(* Logix 5000 AddOnInstructionDefinition export AOI_MOXA_SWITCH_28P_v1_1; software revision 20.01 *)

TYPE MOXA_Ethernet_Link_Object :   // class 0xf6
STRUCT
   Interface_Speed : DINT;   // Interface speed currently in use. Speed in Mbps (e.g., 0, 10, 100, 1000, etc.)
   Interface_Flags : MOXA_Interface_Object_Flags;   // Interface status flags
   Physical_Address : SINT[6];   // MAC layer address
   InOctets : DINT;   // Octets received on the interface
   InUcastPackets : DINT;   // Unicast packets received on the interface
   InNucastPackets : DINT;   // Non-unicast packets received on the interface
   InDiscards : DINT;   // Inbound packets received on the interface but discarded
   InErrors : DINT;   // Inbound packets that contain errors (does not include In Discards)
   InUnknownProtos : DINT;   // Inbound packets with unknown protocol.
   OutOctets : DINT;   // Octets sent on the interface
   OutUcastPackets : DINT;   // Unicast packets sent on the interface
   OutNucastPackets : DINT;   // Non-unicast packets sent on the interface
   OutDiscards : DINT;   // Outbound packets discarded
   OutErrors : DINT;   // Outbound packets that contain errors
   Alignment_Errors : DINT;   // Frames received that are not an integral number of octets in length
   FCS_Errors : DINT;   // Frames received that do not pass the FCS check
   Single_Collisions : DINT;   // Successfully transmitted frames which experienced exactly one collision
   Multiple_Collisions : DINT;   // Successfully transmitted frames which experienced more than one collision
   SQE_Test_Errors : DINT;   // Number of times SQE test error message is generated
   Deferred_Transmissions : DINT;   // Frames for which first transmission attempt is delayed because the medium is busy
   Late_Collisions : DINT;   // Number of times a collision is detected later than 512 bit- times into the transmission of a packet
   Excessive_Collisions : DINT;   // Frames for which transmission fails due to excessive collisions
   MAC_Transmit_Errors : DINT;   // Frames for which transmission fails due to an internal MAC sublayer transmit error
   Carrier_Sense_Errors : DINT;   // Times that the carrier sense condition was lost or never asserted when attempting to transmit a frame
   Frame_Too_Long : DINT;   // Frames received tha exceed the maximum permitted frame size.
   MAC_Receive_Errors : DINT;   // Frames for which reception on an interface fails due to an internal MAC sublayer receive error
   Control_Bits : INT;   // Bit 0 Auto-negotiate Bit 1: Forced Duplex Mode Bit 2-15: Reserved.
   Forced_Interface_Speed : INT;   // Speed at which the interface shall be forced to operate. Speed in Mbps (10, 100, 1000, etc.)
   Interface_Label : STRING;   // Port Description
   Capability_Bits : DINT;
   Speed_Duplex_Array : SINT;   // Number of elements
   Interface_Speed_Duplex_Capbility : MOXA_Interface_Capability[4];
   HC_InOctets : LINT;   // The total number of octets received on the interface. This counter is a 64-bit version of In Octets.
   HC_InUcastPkts : LINT;   // Unicast packets received on the interface. This counter is a 64-bit version of In Ucast Packets.
   HC_InMulticastPkts : LINT;   // Multicast packets received on the interface.
   HC_InBroadcastPkts : LINT;   // Broadcast packets received on the interface.
   HC_OutOctets : LINT;   // Octets sent on the interface. This counter is a 64-bit version of Out Octets.
   HC_OutUcastPkts : LINT;   // Unicast packets sent on the interface. This counter is a 64-bit version of Out Ucast Packets.
   HC_OutMulticastPkts : LINT;   // Multicast packets sent on the interface.
   HC_OutBroadcastPkts : LINT;   // Broadcast packets sent on the interface.
   HC_StatsAlignmentErrors : LINT;   // Frames received that are not an integral number of octets in length and do not pass the FCS check. This counter is a 64-bit version of Alignment Errors.
   HC_StatsFCSErrors : LINT;   // Frames received that are an integral number of octets in length but do not pass the FCS check. This counter is a 64-bit version of FCS Errors.
   HC_StatsInternalMacTransmitErrors : LINT;   // Frames for which transmission fails due to an internal MAC sublayer transmit error. This counter is a 64-bit version of MAC Transmit Errors.
   HC_StatsFrameTooLongs : LINT;   // Frames received that exceed the maximum permitted frame size. This counter is a 64-bit version of Frame Too Long Errors.
   HC_StatsInternalMacReceiveErrors : LINT;   // Frames for which reception on an interface fails due to an internal MAC sublayer receive error. This counter is a 64-bit version of MAC Receive Errors.
   HC_StatsSymbolErrors : LINT;   // Number of times there was an invalid data symbol on the media when a valid carrier was present.
   Port_State : SINT;   // Switch port state. Value 1 = Disable Value 2 = Blocking Value 3 = Listening Value 4 = Learning Value 5 = Forwarding Value 6 = Broken
   Media_Type : STRING;   // Port media type. Ex: "1000TX,RJ45"
   Traffic_Storm_Control : SINT;   // Traffic storm control enable. Bit 0: Broadcast storm control Bit 1: Multicast storm control Bit 2: DLF storm control
   Port_On_Event : SINT;   // Registered port for port on event notification. 0 = Unregistered. 1 = Registered.
   Port_Off_Event : SINT;   // Registered port for port off event notification. 0 = Unregistered. 1 = Registered.
   Port_Shutdown_by_PSEC_Event : SINT;   // Registered port for port shut down by Port Security event notification. 0 = Unregistered. 1 = Registered.
   Port_Shutdown_by_Rate_Limit_Event : SINT;   // Registered port for port shut down by Rate Limit event notification. 0 = Unregistered. 1 = Registered.
   Port_Recovered_by_Rate_Limit_Event : SINT;   // Registered port for port recovered by Rate Limit event notification. 0 = Unregistered. 1 = Registered.
   Fiber_Check_Warning_Event : SINT;   // Registered port for fiber check warning event notification. 0 = Unregistered. 1 = Registered.
END_STRUCT
END_TYPE

TYPE MOXA_TCPIP_Interface_Object :   // class 0xf5
STRUCT
   Status : DINT; {access Read Only}   // Interface Status
   Configuration_Capability : DINT;   // Interface capability flags
   Configuration_Control : DINT;   // Interface control flags
   Path_Size : INT;   // Size of Path
   Object_Path : DINT;   // Logical segments identifying the physical link object
   IP_Address : DINT;   // The device’s IP address.
   Network_Mask : DINT;   // The device’s network mask
   Gateway_Address : DINT;   // Default gateway address
   Name_Server_1 : DINT;   // Primary name server
   Name_Server_2 : DINT;   // Secondary name server
   Domain_Name : STRING;   // Default domain name
   Host_Name : STRING;   // Host Name
   Encapsulation_InactivityTimeout : INT;   // Number of seconds of inactivity before TCP connection is closed.
END_STRUCT
END_TYPE

TYPE MOXA_Interface_Capability :   // Indication of capabilities of the interface
STRUCT
   Interface_Speed_Capbility : INT;   // Interface speed currently in use. Speed in Mbps (e.g., 0, 10, 100, 1000, etc.)
   Interface_Duplex_Mode : SINT;   // 0=half duplex, 1=full duplex
END_STRUCT
END_TYPE

TYPE MOXA_String_32 :   // string type; Display the ip address, network mask, MAC address
STRUCT
   LEN : DINT;
   DATA : SINT[32];
END_STRUCT
END_TYPE

TYPE MOXA_HMI_Set_Object :
STRUCT
   Select_Port : INT;   // current port select on FT View
   Reset_to_default : SINT;   // Reboot and reset to default. 0 = Reserved. 1 = Reboot the device 2 = Reset to default
   Reset_MIB_Counter : SINT;   // Reset MIB counters. Any value indicates to reset port MIB counter.
   Speed_Duplex : SINT;
   Enter_Port_Setting : BOOL;   // Ready for port setting
   Enter_Reset_Setting : BOOL;   // Ready for resetting.
END_STRUCT
END_TYPE

TYPE MOXA_Interface_Object_Flags :   // reference to Ethernet Link object
STRUCT
   Link_Status : BOOL;   // 0-inactive, 1-active
   Duplex : BOOL;   // 0-half, 1-full
   Negotiation_Status_1 : BOOL;
   Negotiation_Status_2 : BOOL;
   Negotiation_Status_3 : BOOL;
   Manual_Setting_Requires_Reset : BOOL;
   Local_Hardware_Fault : BOOL;
END_STRUCT
END_TYPE

TYPE MOXA_Base_Switch_Object :   // calss 0x51
STRUCT
   Device_Up_Time : DINT;   // Time since device was powered up.
   Total_Port_Count : DINT;   // Number of physical available ports.
   System_Firmware_Version : STRING;   // Human readable representation of System Firmware Version. Maximum length is 32 characters.
   Power_Source : INT;   // Status of switch power source.
   Port_Mask_Size : INT;   // Number of DWORDs in port array attributes. Minimum = 4, supporting 128 ports.
   Existing_Port : DINT[4];   // Switch existing port. 0 = Port Absent 1 = Port Present
   Global_Port_Admin_State : DINT[4];   // Port Admin State. 0 = Port Disabled, 1 = Port Enabled
   Global_Port_Link_Status : DINT[4];   // Ports Link Status. 0 = Link Inactive (Down), 1 = Link Active (Up) Bit 0-31: Port 0-31 Link status.
END_STRUCT
END_TYPE

TYPE MOXA_Object_Data :   // This UDT contains various information that appears on an HMI display. Some information applies to the switch, and some applies to the selected port (copied, or derived from, the port Ethernet_Link data) because FactoryTalk can not access array elements.
STRUCT
   Firmware_Version : STRING;   // Show system firmware version.
   IP_Address : MOXA_String_32;
   Network_Mask : MOXA_String_32;
   MAC_Address : MOXA_String_32;
END_STRUCT
END_TYPE

TYPE MOXA_String_1024 :   // string type
STRUCT
   LEN : DINT;
   DATA : SINT[1024];
END_STRUCT
END_TYPE

TYPE MOXA_Switch_Parameter :
STRUCT
   Switch_Input : SINT[18];   // recieve message from switch
   Switch_Output : SINT[16];   // send message to switch
   Switch_Identity : MOXA_Identity_Object;
   Switch_Base_Switch : MOXA_Base_Switch_Object;
   Switch_TCPIP_Interface : MOXA_TCPIP_Interface_Object;
   Switch_Ethernet_Link : MOXA_Ethernet_Link_Object[29];
   Switch_Moxa_Networking : MOXA_Networking_Object;
   Switch_HMI_Set : MOXA_HMI_Set_Object;
   Switch_Data : MOXA_Object_Data;
END_STRUCT
END_TYPE

TYPE MOXA_Networking_Object :   // class 0x404
STRUCT
   CPU_Usage : SINT;   // Percentage of CPU usage
   L2_Redundancy : SINT;   // Bit 0: RSTP Bit 1: MSTP Bit 2: Turbo Chain Bit 3: Turbo Ring v2 Bit 4: Dual-Homing Bit 5: MRP
   Relay_Alarm_Status : SINT;   // Relay alarm event-triggered status
   Cold_Start : SINT;   // System cold start event notification.
   Warm_Start : SINT;   // System warm start event notification.
   Redundant_Port_Health_Check_Fail : SINT;   // Redundant port health check fail.
   PD_Over_Current : SINT;   // Current of port has exceeded the safety limit.
   PD_No_Response : SINT;   // Port device is not responding to the PD failure check.
   Power_On : SINT;   // Power supply on event notification.
   Power_Off : SINT;   // Power supply off event notification.
   DI_On : SINT;   // Digital input on event notification.
   DI_Off : SINT;   // Digital input off event notification.
   Port_On : SINT;   // Port link up event notification.
   Port_Off : SINT;   // Port link down event notification.
   Port_Shutdown_by_PSEC : SINT;   // Port shutdown by Port Security event notification.
   Port_Shutdown_by_Rate_Limit : SINT;   // Port shutdown by Rate Limit event notification.
   Port_Recovered_by_Rate_Limit : SINT;   // Port recovered by Rate Limit event notification.
   Fiber_Check_Warning : SINT;   // Fiber check warning event notification.
   Relay_Alarm_Cut_Off : SINT;   // Cut off the relay alarm
   Reset_Mib_Counter : SINT;   // Reset port MIB counters.
   Reset_Device : SINT;   // Reboot and reset to default. Value 0 = Reserved. Value 1 = Reboot the device. Value 2 = Reset to default .
END_STRUCT
END_TYPE

TYPE MOXA_Identity_Object :   // class 0x01
STRUCT
   Vendor_ID : INT;   // ODVA Vendor ID. Moxa = 0x3DF
   Device_Type : INT;   // 0x2C, "Managed Ethernet Switch"
   Product_Code : INT;   // Ex: RKS-G4028-4GT-HV = 0x1301
   Major_Revision : SINT;   // Major revision of the item the Identity Object represents
   Minor_Revision : SINT;   // Minor revision of the item the Identity Object represents
   Status : INT;   // Summary status of device
   Serial_Number : DINT;   // Serial number of device
   Product_Name : STRING; {access Read Only}   // Human readable identification. Switch model number. RKS-G4028-4GT-HV
   Assigned_Name : MOXA_String_1024;   // User assigned switch name.
   Geographic_Location : MOXA_String_1024;   // This is the user assigned switch location.
END_STRUCT
END_TYPE

ADD_ON_INSTRUCTION AOI_MOXA_SWITCH_28P_v1_1   (* revision 1.1, vendor MOXA Corporation *)
// The AOI of MOXA switch
// Copyright MOXA Corp. 2024 Version: 1.1
// Date: Feb 6, 2024
VAR_IN_OUT
   Switch_Input : SINT[18]; {required}   // The module defined array representing the input assembly.
   Switch_Output : SINT[16]; {required}   // The module defined array representing the output assembly.
   Switch_Parameter : MOXA_Switch_Parameter; {required}
        .SWITCH_HMI_SET.SELECT_PORT   // Currently selected port
   Get_AllMessage : MESSAGE; {required}   // Message to retrieve parameters from CIP object what service is Get_Attributes_All.
   Get_SingleMessage : MESSAGE; {required}   // Message to retrieve parameters from CIP object what service is Get_Attribute_Single
   Set_SingleMessage : MESSAGE; {required}   // Message to send parameters to CIP object what service is Set_Attibute_Single.
   Set_Data : INT[2]; {required}
   storage : SINT[200]; {required}   // Retrieve data buffers from CIP object what service is Get_Attributes_All.
   storage_single : SINT[200]; {required}   // Retrieve data buffers from CIP object what service is Get_Attribute_Single.
   tcpip_storage : SINT[200]; {required}
   Get_TCPIP_AllMessage : MESSAGE; {required}
END_VAR
VAR
   SelectCounter : COUNTER := (PRE := 371); {access None}
   timer_explicit : TIMER := (PRE := 600); {access None}
   timer_io : TIMER := (PRE := 50); {access None}
   AttributeSelectCounter : DINT; {access None}
   portnum_index : SINT; {access None}
   Max_Port : SINT := 28; {access None}
   Min_Port : SINT := 1; {access None}
   String_Len : DINT; {access None}
   Update_Flag : BOOL; {access None}   // Update flags. Start to read message.
   ONS_GetSingle : BOOL; {access None}
   ONS_GetAll : BOOL; {access None}
   Data_Offset : DINT; {access None}   // Add string length bytes to Data_Offset
   Network_Mask_OctetArray : DINT[4]; {access None}
   IP_Address_OctetArray : DINT[4]; {access None}
   Network_Mask_StringArray : STRING[4]; {access None}
   IP_Address_StringArray : STRING[4]; {access None}
   punctuation_marks : STRING; {access None}   // Add punctuation into string. ex: ".", "-"
   MAC_StringArray : STRING[12]; {access None}
   temp_data : DINT; {access None}
   ONS_TCPIP_GetAll : BOOL; {access None}
   Attribute_Num : DINT; {access None}
   MAC_OctetArray : DINT[12]; {access None}
   b_SetPortDuplex : BOOL; {access None}
   b_SetMSG : BOOL; {access None}
   Forced_Interface_Speed : INT; {access None}
   Control_Bits : INT; {access None}
   remainder : DINT; {access None}   // MOD value of string length for aligning pad byte
END_VAR

ROUTINE Logic   (* ladder *)
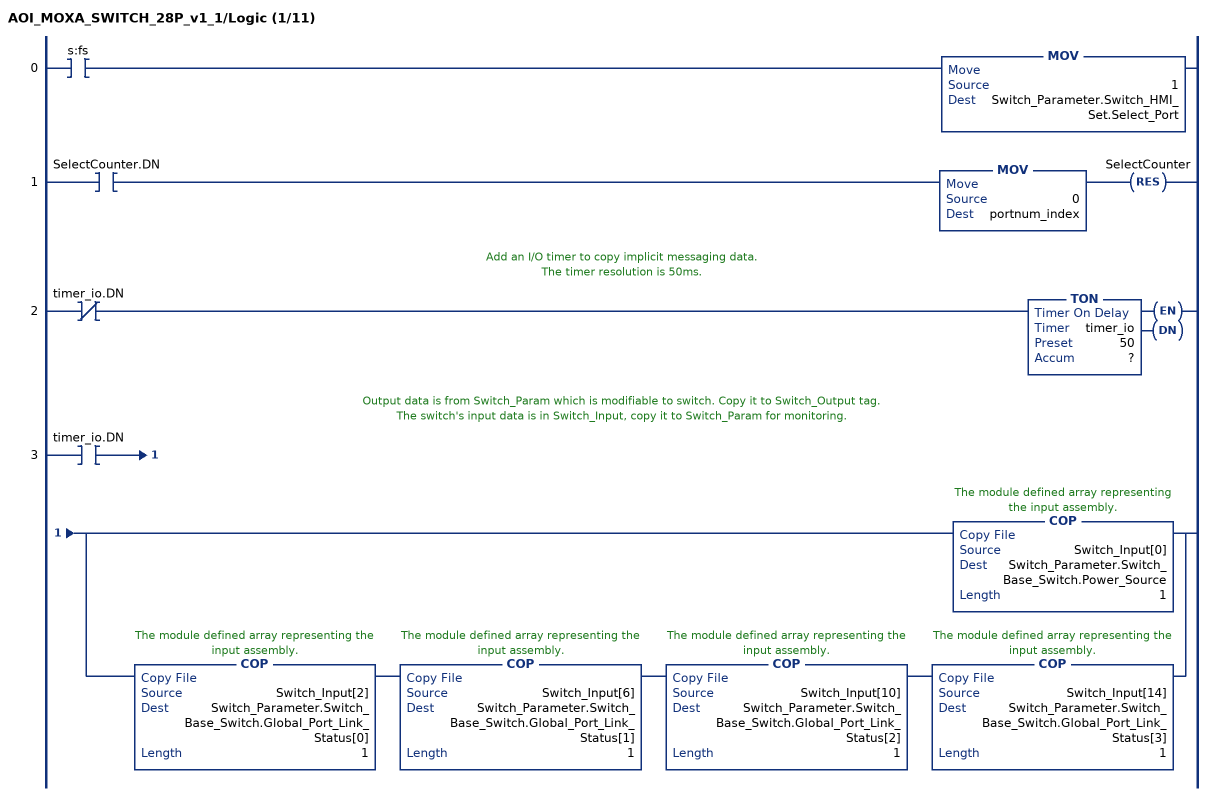
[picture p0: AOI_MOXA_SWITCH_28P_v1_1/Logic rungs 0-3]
   0: XIC(s:fs)MOV(1,Switch_Parameter.Switch_HMI_Set.Select_Port);
   1: XIC(SelectCounter.DN)MOV(0,portnum_index)RES(SelectCounter);
   // Add an I/O timer to copy implicit messaging data.
   // The timer resolution is 50ms.
   2: XIO(timer_io.DN)TON(timer_io,?,?);
   // Output data is from Switch_Param which is modifiable to switch. Copy it to Switch_Output tag.
   // The switch's input data is in Switch_Input, copy it to Switch_Param for monitoring.
   3: XIC(timer_io.DN)[COP(Switch_Input[0],Switch_Parameter.Switch_Base_Switch.Power_Source,1) ,COP(Switch_Input[2],Switch_Parameter.Switch_Base_Switch.Global_Port_Link_Status[0],1) COP(Switch_Input[6],Switch_Parameter.Switch_Base_Switch.Global_Port_Link_Status[1],1) COP(Switch_Input[10],Switch_Parameter.Switch_Base_Switch.Global_Port_Link_Status[2],1) COP(Switch_Input[14],Switch_Parameter.Switch_Base_Switch.Global_Port_Link_Status[3],1) ];
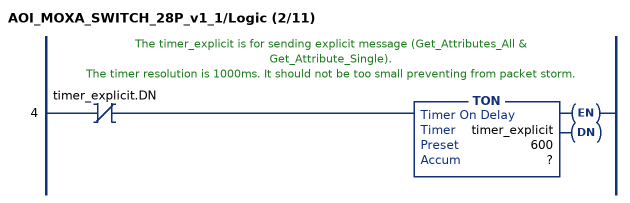
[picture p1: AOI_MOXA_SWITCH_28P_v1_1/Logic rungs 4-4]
   // The timer_explicit is for sending explicit message (Get_Attributes_All & Get_Attribute_Single).
   // The timer resolution is 1000ms. It should not be too small preventing from packet storm.
   4: XIO(timer_explicit.DN)TON(timer_explicit,?,?);
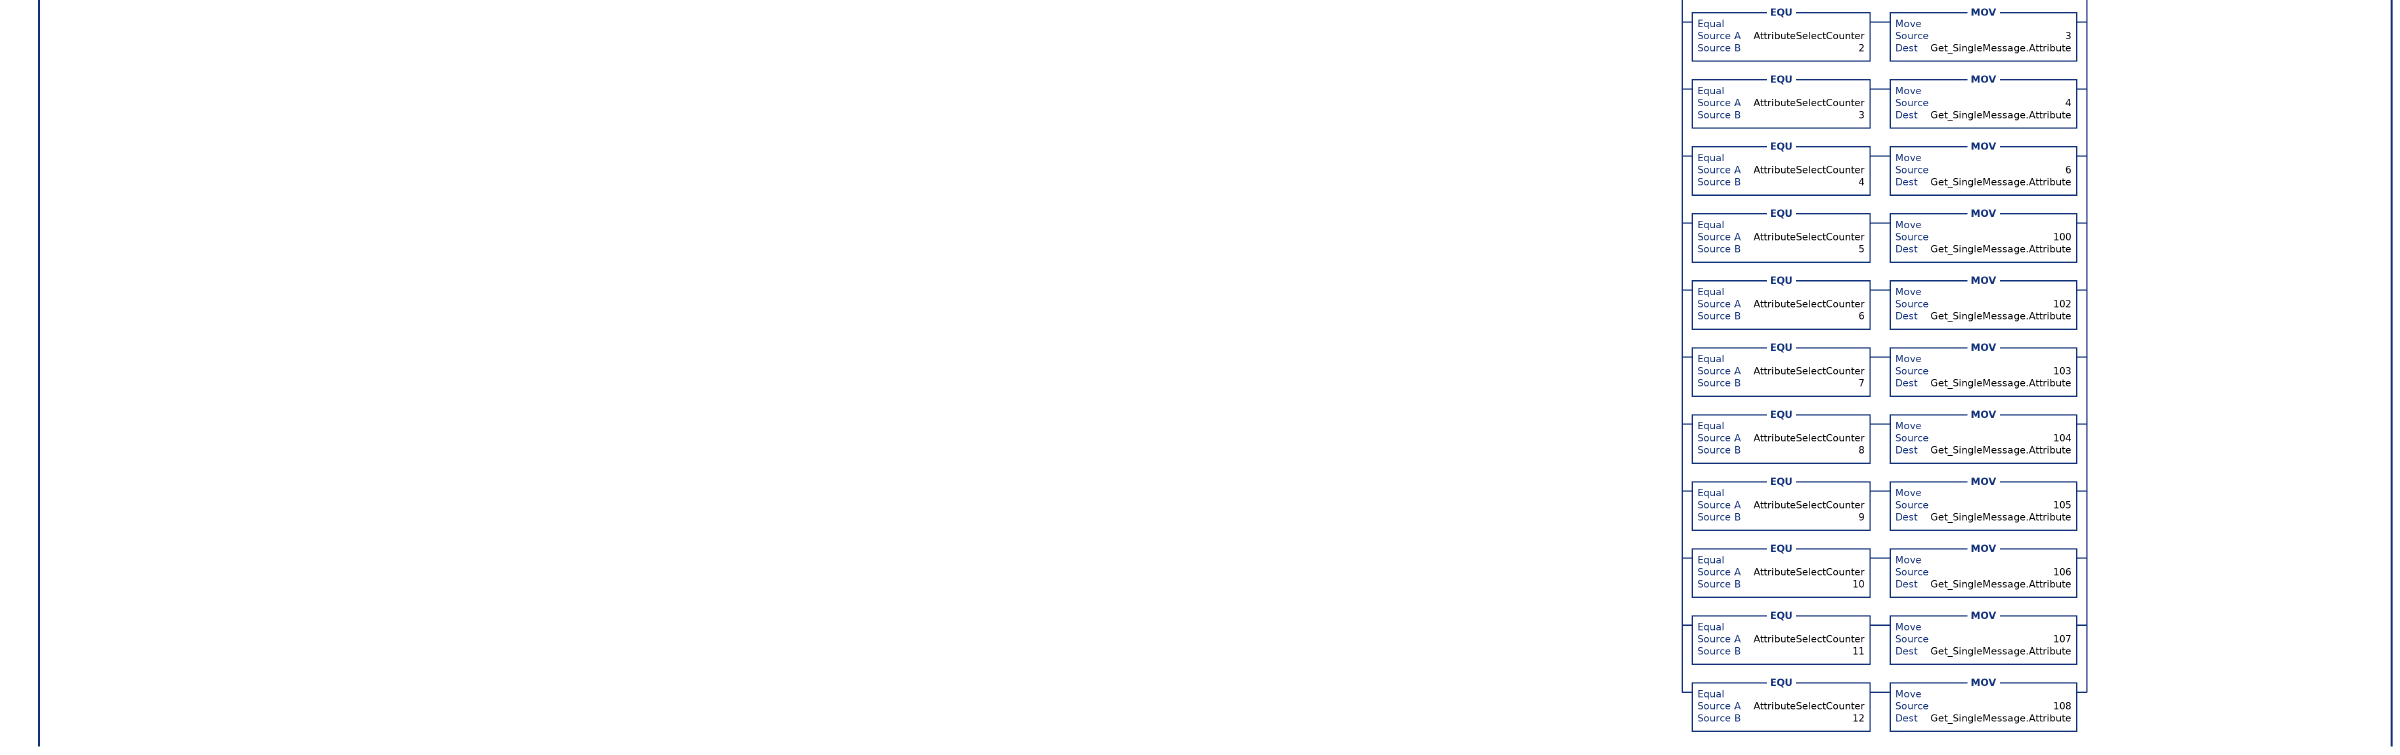
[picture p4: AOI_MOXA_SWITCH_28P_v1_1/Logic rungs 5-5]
   // If SelectCounter.ACC== 1, send GAA of Identity object (Class ID = 0x01).
   // If SelectCounter.ACC== 2, send GAA of TCP/IP object (Class ID = 0xF5).
   // If SelectCounter.ACC== 3-10, send GAS of Base Switch object (class ID = 0x51) for Attributes 1-8.
   // If SelectCounter.ACC== 11-19, send GAS of Vendor object (class ID = 0x404) for Attributes 1-3 & 13-18.
   // If SelectCounter.ACC==??, snd GAS of Ethernet Link object(Class ID = 0xF6)
   5: XIC(timer_explicit.DN)CTU(SelectCounter,?,?)[EQU(SelectCounter.ACC,1) MOV(1,Get_AllMessage.Class) MOV(1,Get_AllMessage.Instance) MOV(1,Get_AllMessage.Attribute) MSG(Get_AllMessage) ,EQU(SelectCounter.ACC,2) MOV(245,Get_TCPIP_AllMessage.Class) MOV(1,Get_TCPIP_AllMessage.Instance) MOV(1,Get_TCPIP_AllMessage.Attribute) MSG(Get_TCPIP_AllMessage) ,XIO(ONS_GetSingle) LIM(3,SelectCounter.ACC,10) OTL(ONS_GetSingle) MOV(SelectCounter.ACC,Attribute_Num) MOV(81,Get_SingleMessage.Class) MOV(1,Get_SingleMessage.Instance) [EQU(Attribute_Num,3) MOV(1,Get_SingleMessage.Attribute) ,EQU(Attribute_Num,4) MOV(2,Get_SingleMessage.Attribute) ,EQU(Attribute_Num,5) MOV(3,Get_SingleMessage.Attribute) ,EQU(Attribute_Num,6) MOV(4,Get_SingleMessage.Attribute) ,EQU(Attribute_Num,7) MOV(5,Get_SingleMessage.Attribute) ,EQU(Attribute_Num,8) MOV(6,Get_SingleMessage.Attribute) ,EQU(Attribute_Num,9) MOV(7,Get_SingleMessage.Attribute) ,EQU(Attribute_Num,10) MOV(8,Get_SingleMessage.Attribute) ] MSG(Get_SingleMessage) ,XIO(ONS_GetSingle) LIM(11,SelectCounter.ACC,19) OTL(ONS_GetSingle) MOV(SelectCounter.ACC,Attribute_Num) MOV(1028,Get_SingleMessage.Class) MOV(1,Get_SingleMessage.Instance) [EQU(Attribute_Num,11) MOV(1,Get_SingleMessage.Attribute) ,EQU(Attribute_Num,12) MOV(2,Get_SingleMessage.Attribute) ,EQU(Attribute_Num,13) MOV(3,Get_SingleMessage.Attribute) ,EQU(Attribute_Num,14) MOV(13,Get_SingleMessage.Attribute) ,EQU(Attribute_Num,15) MOV(14,Get_SingleMessage.Attribute) ,EQU(Attribute_Num,16) MOV(15,Get_SingleMessage.Attribute) ,EQU(Attribute_Num,17) MOV(16,Get_SingleMessage.Attribute) ,EQU(Attribute_Num,18) MOV(17,Get_SingleMessage.Attribute) ,EQU(Attribute_Num,19) MOV(18,Get_SingleMessage.Attribute) ] MSG(Get_SingleMessage) ,XIO(ONS_GetSingle) LIM(20,SelectCounter.ACC,371) OTL(ONS_GetSingle) MOV(SelectCounter.ACC,Attribute_Num) SUB(Attribute_Num,20,AttributeSelectCounter) DIV(AttributeSelectCounter,13,temp_data) ADD(temp_data,1,portnum_index) MOD(AttributeSelectCounter,13,AttributeSelectCounter) MOV(246,Get_SingleMessage.Class) MOV(portnum_index,Get_SingleMessage.Instance) [EQU(AttributeSelectCounter,0) MOV(1,Get_SingleMessage.Attribute) ,EQU(AttributeSelectCounter,1) MOV(2,Get_SingleMessage.Attribute) ,EQU(AttributeSelectCounter,2) MOV(3,Get_SingleMessage.Attribute) ,EQU(AttributeSelectCounter,3) MOV(4,Get_SingleMessage.Attribute) ,EQU(AttributeSelectCounter,4) MOV(6,Get_SingleMessage.Attribute) ,EQU(AttributeSelectCounter,5) MOV(100,Get_SingleMessage.Attribute) ,EQU(AttributeSelectCounter,6) MOV(102,Get_SingleMessage.Attribute) ,EQU(AttributeSelectCounter,7) MOV(103,Get_SingleMessage.Attribute) ,EQU(AttributeSelectCounter,8) MOV(104,Get_SingleMessage.Attribute) ,EQU(AttributeSelectCounter,9) MOV(105,Get_SingleMessage.Attribute) ,EQU(AttributeSelectCounter,10) MOV(106,Get_SingleMessage.Attribute) ,EQU(AttributeSelectCounter,11) MOV(107,Get_SingleMessage.Attribute) ,EQU(AttributeSelectCounter,12) MOV(108,Get_SingleMessage.Attribute) ] MSG(Get_SingleMessage) ];
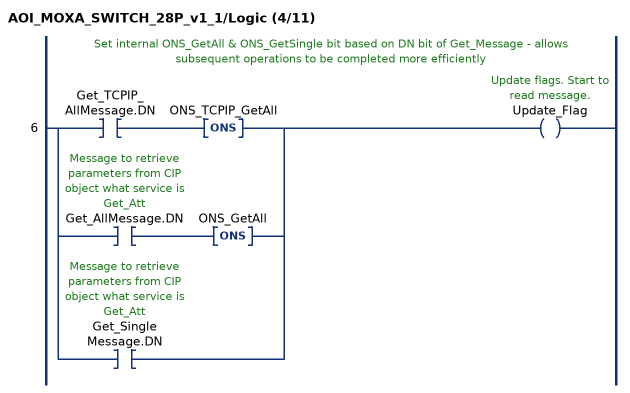
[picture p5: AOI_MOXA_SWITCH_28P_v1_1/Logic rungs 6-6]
   // Set internal ONS_GetAll & ONS_GetSingle bit based on DN bit of Get_Message - allows subsequent operations to be completed more efficiently
   6: [XIC(Get_TCPIP_AllMessage.DN) ONS(ONS_TCPIP_GetAll) ,XIC(Get_AllMessage.DN) ONS(ONS_GetAll) ,XIC(Get_SingleMessage.DN) ]OTE(Update_Flag);
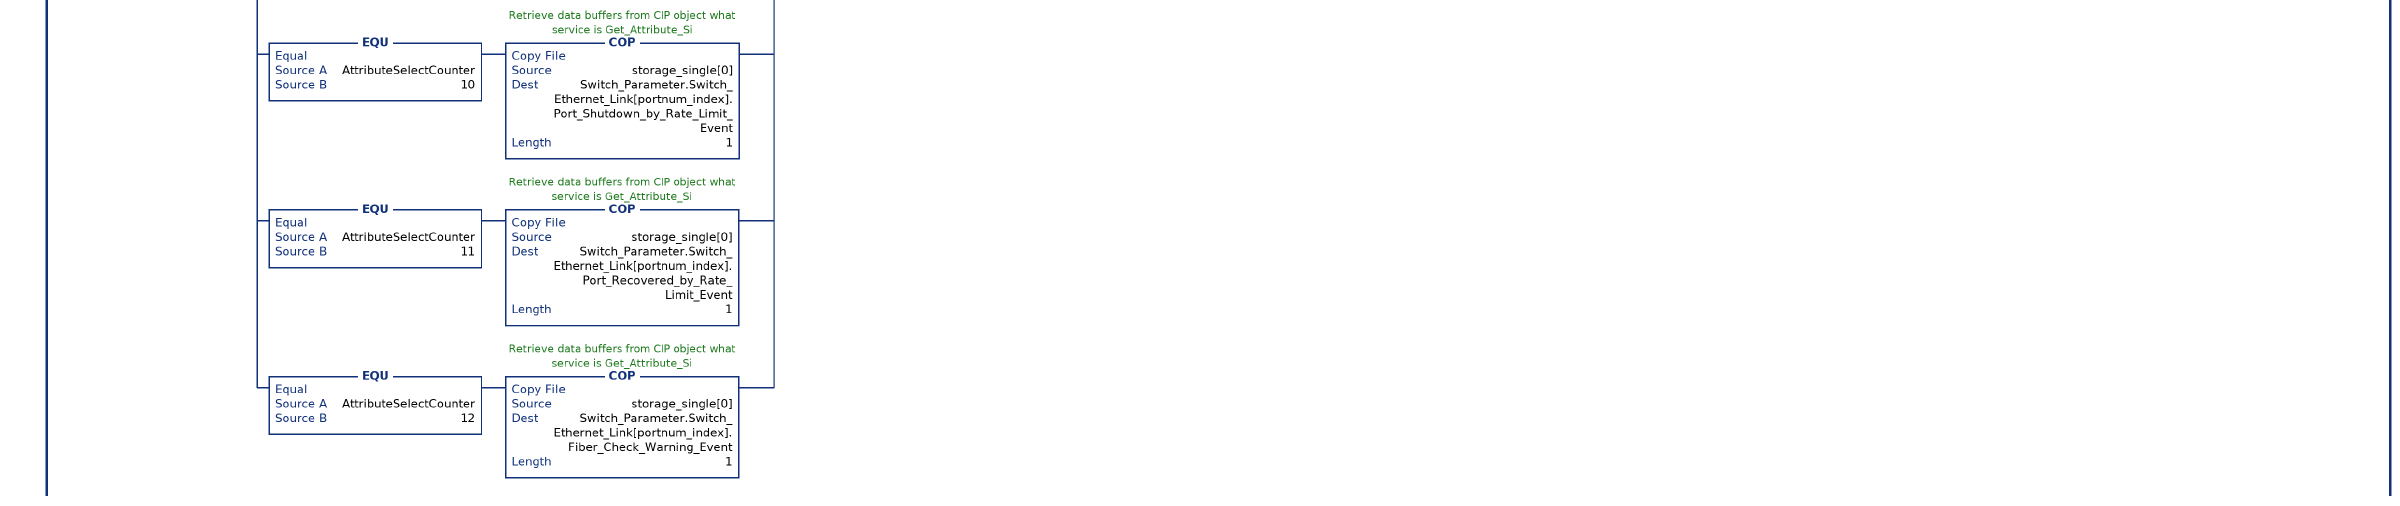
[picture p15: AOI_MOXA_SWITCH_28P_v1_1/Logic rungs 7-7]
   // Copy results of Get Attribute All
   // If counter = 1: Identity Object - Class 1, Instance 1, Attribute 1
   // If counter = 2: TCP/IP Interface Object, Class 245, Instance 1, Attribute 1
   // If counter = 3 : Vendor Object, Class 1028, Instance 1, Attribute 1
   // If counter = 4~15 : EtherNet Link Object, Class 246, Instance 1 to 12 , Attribute 1 - EthernetLink[1-12]
   7: XIC(Update_Flag)[EQU(SelectCounter.ACC,1) [COP(storage[0],Switch_Parameter.Switch_Identity.Vendor_ID,1) ,COP(storage[2],Switch_Parameter.Switch_Identity.Device_Type,1) ,COP(storage[4],Switch_Parameter.Switch_Identity.Product_Code,1) ,COP(storage[6],Switch_Parameter.Switch_Identity.Major_Revision,1) ,COP(storage[7],Switch_Parameter.Switch_Identity.Minor_Revision,1) ,COP(storage[8],Switch_Parameter.Switch_Identity.Status,1) ,COP(storage[10],Switch_Parameter.Switch_Identity.Serial_Number,1) ,MOV(storage[14],String_Len) MOV(String_Len,Switch_Parameter.Switch_Identity.Product_Name.LEN) FLL(0,Switch_Parameter.Switch_Identity.Product_Name.DATA[0],String_Len) COP(storage[15],Switch_Parameter.Switch_Identity.Product_Name.DATA[0],String_Len) ] ,EQU(SelectCounter.ACC,2) [COP(tcpip_storage[0],Switch_Parameter.Switch_TCPIP_Interface.Status,1) ,COP(tcpip_storage[4],Switch_Parameter.Switch_TCPIP_Interface.Configuration_Capability,1) ,COP(tcpip_storage[8],Switch_Parameter.Switch_TCPIP_Interface.Configuration_Control,1) ,COP(tcpip_storage[12],Switch_Parameter.Switch_TCPIP_Interface.Path_Size,1) ,COP(tcpip_storage[14],Switch_Parameter.Switch_TCPIP_Interface.Object_Path,1) ,COP(tcpip_storage[18],Switch_Parameter.Switch_TCPIP_Interface.IP_Address,1) ,COP(tcpip_storage[22],Switch_Parameter.Switch_TCPIP_Interface.Network_Mask,1) ,COP(tcpip_storage[26],Switch_Parameter.Switch_TCPIP_Interface.Gateway_Address,1) ,COP(tcpip_storage[30],Switch_Parameter.Switch_TCPIP_Interface.Name_Server_1,1) ,COP(tcpip_storage[34],Switch_Parameter.Switch_TCPIP_Interface.Name_Server_2,1) ,MOV(38,Data_Offset) MOV(tcpip_storage[Data_Offset],String_Len) MOV(String_Len,Switch_Parameter.Switch_TCPIP_Interface.Domain_Name.LEN) ADD(2,Data_Offset,Data_Offset) FLL(0,Switch_Parameter.Switch_TCPIP_Interface.Domain_Name.DATA[0],82) COP(tcpip_storage[Data_Offset],Switch_Parameter.Switch_TCPIP_Interface.Domain_Name.DATA[0],String_Len) ADD(String_Len,Data_Offset,Data_Offset) MOD(String_Len,2,remainder) EQU(remainder,1) ADD(Data_Offset,remainder,Data_Offset) ,MOV(tcpip_storage[Data_Offset],String_Len) MOV(String_Len,Switch_Parameter.Switch_TCPIP_Interface.Host_Name.LEN) ADD(2,Data_Offset,Data_Offset) FLL(0,Switch_Parameter.Switch_TCPIP_Interface.Host_Name.DATA[0],82) COP(tcpip_storage[Data_Offset],Switch_Parameter.Switch_TCPIP_Interface.Host_Name.DATA[0],String_Len) ADD(String_Len,Data_Offset,Data_Offset) MOD(String_Len,2,remainder) EQU(remainder,1) ADD(Data_Offset,remainder,Data_Offset) ,ADD(Data_Offset,52,Data_Offset) COP(tcpip_storage[Data_Offset],Switch_Parameter.Switch_TCPIP_Interface.Encapsulation_InactivityTimeout,1) ] ,LIM(3,Attribute_Num,10) [EQU(Attribute_Num,3) COP(storage_single[0],Switch_Parameter.Switch_Base_Switch.Device_Up_Time,1) ,EQU(Attribute_Num,4) COP(storage_single[0],Switch_Parameter.Switch_Base_Switch.Total_Port_Count,1) ,EQU(Attribute_Num,5) MOV(storage_single[0],Switch_Parameter.Switch_Base_Switch.System_Firmware_Version.LEN) FLL(0,Switch_Parameter.Switch_Base_Switch.System_Firmware_Version.DATA[0],82) COP(storage_single[1],Switch_Parameter.Switch_Base_Switch.System_Firmware_Version.DATA[0],Switch_Parameter.Switch_Base_Switch.System_Firmware_Version.LEN) ,EQU(Attribute_Num,6) COP(storage_single[0],Switch_Parameter.Switch_Base_Switch.Power_Source,1) ,EQU(Attribute_Num,7) COP(storage_single[0],Switch_Parameter.Switch_Base_Switch.Port_Mask_Size,1) ,EQU(Attribute_Num,8) COP(storage_single[0],Switch_Parameter.Switch_Base_Switch.Existing_Port[0],4) ,EQU(Attribute_Num,9) COP(storage_single[0],Switch_Parameter.Switch_Base_Switch.Global_Port_Admin_State[0],4) ,EQU(Attribute_Num,10) COP(storage_single[0],Switch_Parameter.Switch_Base_Switch.Global_Port_Link_Status[0],4) ] OTU(ONS_GetSingle) ,LIM(11,Attribute_Num,19) [EQU(Attribute_Num,11) COP(storage_single[0],Switch_Parameter.Switch_Moxa_Networking.CPU_Usage,1) ,EQU(Attribute_Num,12) COP(storage_single[0],Switch_Parameter.Switch_Moxa_Networking.L2_Redundancy,1) ,EQU(Attribute_Num,13) COP(storage_single[0],Switch_Parameter.Switch_Moxa_Networking.Relay_Alarm_Status,1) ,EQU(Attribute_Num,14) COP(storage_single[0],Switch_Parameter.Switch_Moxa_Networking.Port_On,1) ,EQU(Attribute_Num,15) COP(storage_single[0],Switch_Parameter.Switch_Moxa_Networking.Port_Off,1) ,EQU(Attribute_Num,16) COP(storage_single[0],Switch_Parameter.Switch_Moxa_Networking.Port_Shutdown_by_PSEC,1) ,EQU(Attribute_Num,17) COP(storage_single[0],Switch_Parameter.Switch_Moxa_Networking.Port_Shutdown_by_Rate_Limit,1) ,EQU(Attribute_Num,18) COP(storage_single[0],Switch_Parameter.Switch_Moxa_Networking.Port_Recovered_by_Rate_Limit,1) ,EQU(Attribute_Num,19) COP(storage_single[0],Switch_Parameter.Switch_Moxa_Networking.Fiber_Check_Warning,1) ] OTU(ONS_GetSingle) ,LIM(20,Attribute_Num,371) [EQU(AttributeSelectCounter,0) COP(storage_single[0],Switch_Parameter.Switch_Ethernet_Link[portnum_index].Interface_Speed,1) ,EQU(AttributeSelectCounter,1) COP(storage_single[0],Switch_Parameter.Switch_Ethernet_Link[portnum_index].Interface_Flags,1) ,EQU(AttributeSelectCounter,2) COP(storage_single[0],Switch_Parameter.Switch_Ethernet_Link[portnum_index].Physical_Address[0],6) ,EQU(AttributeSelectCounter,3) [COP(storage_single[0],Switch_Parameter.Switch_Ethernet_Link[portnum_index].InOctets,1) ,COP(storage_single[4],Switch_Parameter.Switch_Ethernet_Link[portnum_index].InUcastPackets,1) ,COP(storage_single[8],Switch_Parameter.Switch_Ethernet_Link[portnum_index].InNucastPackets,1) ,COP(storage_single[12],Switch_Parameter.Switch_Ethernet_Link[portnum_index].InDiscards,1) ,COP(storage_single[16],Switch_Parameter.Switch_Ethernet_Link[portnum_index].InErrors,1) ,COP(storage_single[20],Switch_Parameter.Switch_Ethernet_Link[portnum_index].InUnknownProtos,1) ,COP(storage_single[24],Switch_Parameter.Switch_Ethernet_Link[portnum_index].OutOctets,1) ,COP(storage_single[28],Switch_Parameter.Switch_Ethernet_Link[portnum_index].OutUcastPackets,1) ,COP(storage_single[32],Switch_Parameter.Switch_Ethernet_Link[portnum_index].OutNucastPackets,1) ,COP(storage_single[36],Switch_Parameter.Switch_Ethernet_Link[portnum_index].OutDiscards,1) ,COP(storage_single[40],Switch_Parameter.Switch_Ethernet_Link[portnum_index].OutErrors,1) ] ,EQU(AttributeSelectCounter,4) [COP(storage_single[0],Switch_Parameter.Switch_Ethernet_Link[portnum_index].Control_Bits,1) ,COP(storage_single[2],Switch_Parameter.Switch_Ethernet_Link[portnum_index].Forced_Interface_Speed,1) ] ,EQU(AttributeSelectCounter,5) COP(storage_single[0],Switch_Parameter.Switch_Ethernet_Link[portnum_index].Port_State,1) ,EQU(AttributeSelectCounter,6) COP(storage_single[0],Switch_Parameter.Switch_Ethernet_Link[portnum_index].Traffic_Storm_Control,1) ,EQU(AttributeSelectCounter,7) COP(storage_single[0],Switch_Parameter.Switch_Ethernet_Link[portnum_index].Port_On_Event,1) ,EQU(AttributeSelectCounter,8) COP(storage_single[0],Switch_Parameter.Switch_Ethernet_Link[portnum_index].Port_Off_Event,1) ,EQU(AttributeSelectCounter,9) COP(storage_single[0],Switch_Parameter.Switch_Ethernet_Link[portnum_index].Port_Shutdown_by_PSEC_Event,1) ,EQU(AttributeSelectCounter,10) COP(storage_single[0],Switch_Parameter.Switch_Ethernet_Link[portnum_index].Port_Shutdown_by_Rate_Limit_Event,1) ,EQU(AttributeSelectCounter,11) COP(storage_single[0],Switch_Parameter.Switch_Ethernet_Link[portnum_index].Port_Recovered_by_Rate_Limit_Event,1) ,EQU(AttributeSelectCounter,12) COP(storage_single[0],Switch_Parameter.Switch_Ethernet_Link[portnum_index].Fiber_Check_Warning_Event,1) ] OTU(ONS_GetSingle) ];
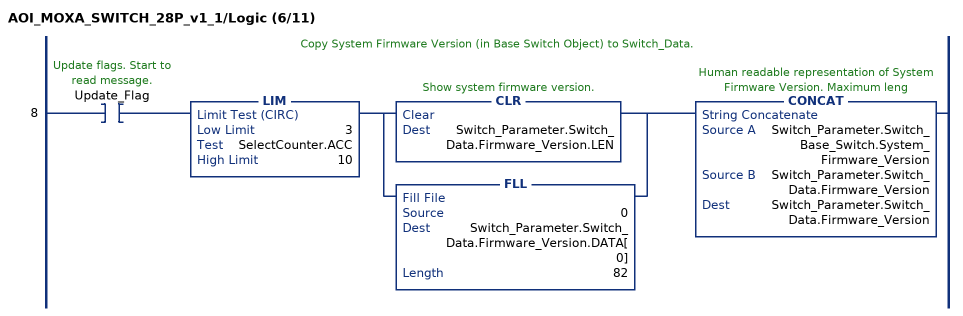
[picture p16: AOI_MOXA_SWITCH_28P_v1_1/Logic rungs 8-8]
   // Copy System Firmware Version (in Base Switch Object) to Switch_Data.
   8: XIC(Update_Flag)LIM(3,SelectCounter.ACC,10)[CLR(Switch_Parameter.Switch_Data.Firmware_Version.LEN) ,FLL(0,Switch_Parameter.Switch_Data.Firmware_Version.DATA[0],82) ]CONCAT(Switch_Parameter.Switch_Base_Switch.System_Firmware_Version,Switch_Parameter.Switch_Data.Firmware_Version,Switch_Parameter.Switch_Data.Firmware_Version);
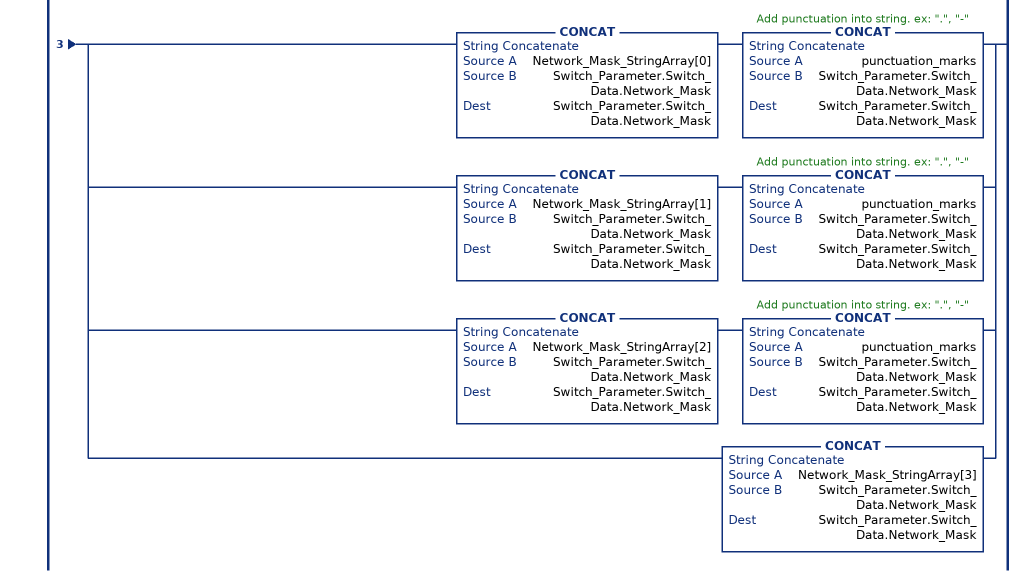
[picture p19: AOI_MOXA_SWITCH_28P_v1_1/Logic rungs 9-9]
   // Convert IP Address and Subnet Mask data type from the Integer to the String.
   9: XIC(Update_Flag)EQU(SelectCounter.ACC,2)[CLR(Switch_Parameter.Switch_Data.IP_Address.LEN) ,FLL(0,Switch_Parameter.Switch_Data.IP_Address.DATA[0],32) ][CLR(Switch_Parameter.Switch_Data.Network_Mask.LEN) ,FLL(0,Switch_Parameter.Switch_Data.Network_Mask.DATA[0],32) ][BTD(Switch_Parameter.Switch_TCPIP_Interface.IP_Address,0,IP_Address_OctetArray[0],0,8) ,BTD(Switch_Parameter.Switch_TCPIP_Interface.IP_Address,8,IP_Address_OctetArray[1],0,8) ,BTD(Switch_Parameter.Switch_TCPIP_Interface.IP_Address,16,IP_Address_OctetArray[2],0,8) ,BTD(Switch_Parameter.Switch_TCPIP_Interface.IP_Address,24,IP_Address_OctetArray[3],0,8) ,BTD(Switch_Parameter.Switch_TCPIP_Interface.Network_Mask,0,Network_Mask_OctetArray[0],0,8) ,BTD(Switch_Parameter.Switch_TCPIP_Interface.Network_Mask,8,Network_Mask_OctetArray[1],0,8) ,BTD(Switch_Parameter.Switch_TCPIP_Interface.Network_Mask,16,Network_Mask_OctetArray[2],0,8) ,BTD(Switch_Parameter.Switch_TCPIP_Interface.Network_Mask,24,Network_Mask_OctetArray[3],0,8) ][DTOS(IP_Address_OctetArray[0],IP_Address_StringArray[0]) ,DTOS(IP_Address_OctetArray[1],IP_Address_StringArray[1]) ,DTOS(IP_Address_OctetArray[2],IP_Address_StringArray[2]) ,DTOS(IP_Address_OctetArray[3],IP_Address_StringArray[3]) ,DTOS(Network_Mask_OctetArray[0],Network_Mask_StringArray[0]) ,DTOS(Network_Mask_OctetArray[1],Network_Mask_StringArray[1]) ,DTOS(Network_Mask_OctetArray[2],Network_Mask_StringArray[2]) ,DTOS(Network_Mask_OctetArray[3],Network_Mask_StringArray[3]) ]MOV(1,punctuation_marks.LEN)MOV(46,punctuation_marks.DATA[0])[CONCAT(IP_Address_StringArray[0],Switch_Parameter.Switch_Data.IP_Address,Switch_Parameter.Switch_Data.IP_Address) CONCAT(punctuation_marks,Switch_Parameter.Switch_Data.IP_Address,Switch_Parameter.Switch_Data.IP_Address) ,CONCAT(IP_Address_StringArray[1],Switch_Parameter.Switch_Data.IP_Address,Switch_Parameter.Switch_Data.IP_Address) CONCAT(punctuation_marks,Switch_Parameter.Switch_Data.IP_Address,Switch_Parameter.Switch_Data.IP_Address) ,CONCAT(IP_Address_StringArray[2],Switch_Parameter.Switch_Data.IP_Address,Switch_Parameter.Switch_Data.IP_Address) CONCAT(punctuation_marks,Switch_Parameter.Switch_Data.IP_Address,Switch_Parameter.Switch_Data.IP_Address) ,CONCAT(IP_Address_StringArray[3],Switch_Parameter.Switch_Data.IP_Address,Switch_Parameter.Switch_Data.IP_Address) ][CONCAT(Network_Mask_StringArray[0],Switch_Parameter.Switch_Data.Network_Mask,Switch_Parameter.Switch_Data.Network_Mask) CONCAT(punctuation_marks,Switch_Parameter.Switch_Data.Network_Mask,Switch_Parameter.Switch_Data.Network_Mask) ,CONCAT(Network_Mask_StringArray[1],Switch_Parameter.Switch_Data.Network_Mask,Switch_Parameter.Switch_Data.Network_Mask) CONCAT(punctuation_marks,Switch_Parameter.Switch_Data.Network_Mask,Switch_Parameter.Switch_Data.Network_Mask) ,CONCAT(Network_Mask_StringArray[2],Switch_Parameter.Switch_Data.Network_Mask,Switch_Parameter.Switch_Data.Network_Mask) CONCAT(punctuation_marks,Switch_Parameter.Switch_Data.Network_Mask,Switch_Parameter.Switch_Data.Network_Mask) ,CONCAT(Network_Mask_StringArray[3],Switch_Parameter.Switch_Data.Network_Mask,Switch_Parameter.Switch_Data.Network_Mask) ];
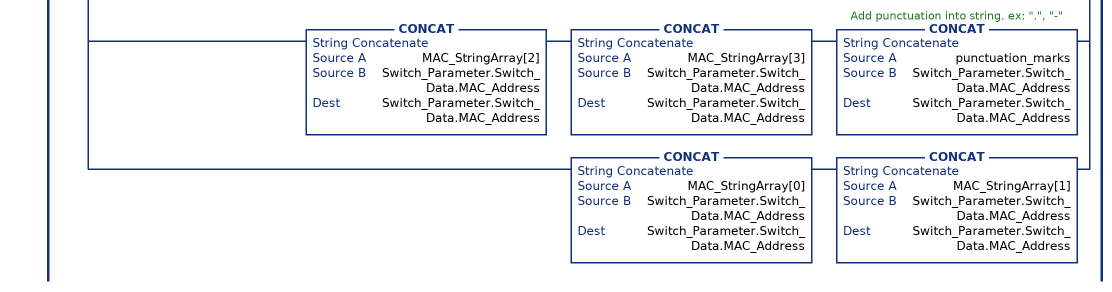
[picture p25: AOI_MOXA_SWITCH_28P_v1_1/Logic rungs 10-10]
   // Convert MAC Address data type from the Integer to the String.
   10: XIC(Update_Flag)LIM(20,SelectCounter.ACC,30)[CLR(Switch_Parameter.Switch_Data.MAC_Address.LEN) ,FLL(0,Switch_Parameter.Switch_Data.MAC_Address.DATA[0],32) ][BTD(Switch_Parameter.Switch_Ethernet_Link[1].Physical_Address[0],0,MAC_OctetArray[0],0,4) BTD(Switch_Parameter.Switch_Ethernet_Link[1].Physical_Address[0],4,MAC_OctetArray[1],0,4) ,BTD(Switch_Parameter.Switch_Ethernet_Link[1].Physical_Address[1],0,MAC_OctetArray[2],0,4) BTD(Switch_Parameter.Switch_Ethernet_Link[1].Physical_Address[1],4,MAC_OctetArray[3],0,4) ,BTD(Switch_Parameter.Switch_Ethernet_Link[1].Physical_Address[2],0,MAC_OctetArray[4],0,4) BTD(Switch_Parameter.Switch_Ethernet_Link[1].Physical_Address[2],4,MAC_OctetArray[5],0,4) ,BTD(Switch_Parameter.Switch_Ethernet_Link[1].Physical_Address[3],0,MAC_OctetArray[6],0,4) BTD(Switch_Parameter.Switch_Ethernet_Link[1].Physical_Address[3],4,MAC_OctetArray[7],0,4) ,BTD(Switch_Parameter.Switch_Ethernet_Link[1].Physical_Address[4],0,MAC_OctetArray[8],0,4) BTD(Switch_Parameter.Switch_Ethernet_Link[1].Physical_Address[4],4,MAC_OctetArray[9],0,4) ,BTD(Switch_Parameter.Switch_Ethernet_Link[1].Physical_Address[5],0,MAC_OctetArray[10],0,4) BTD(Switch_Parameter.Switch_Ethernet_Link[1].Physical_Address[5],4,MAC_OctetArray[11],0,4) ][[LIM(0,MAC_OctetArray[0],9) DTOS(MAC_OctetArray[0],MAC_StringArray[0]) ,LIM(10,MAC_OctetArray[0],15) [MOV(1,MAC_StringArray[0].LEN) ,CPT(MAC_StringArray[0].DATA[0],MAC_OctetArray[0]+55) ] ] ,[LIM(0,MAC_OctetArray[1],9) DTOS(MAC_OctetArray[1],MAC_StringArray[1]) ,LIM(10,MAC_OctetArray[1],15) [MOV(1,MAC_StringArray[1].LEN) ,CPT(MAC_StringArray[1].DATA[0],MAC_OctetArray[1]+55) ] ] ,[LIM(0,MAC_OctetArray[2],9) DTOS(MAC_OctetArray[2],MAC_StringArray[2]) ,LIM(10,MAC_OctetArray[2],15) [MOV(1,MAC_StringArray[2].LEN) ,CPT(MAC_StringArray[2].DATA[0],MAC_OctetArray[2]+55) ] ] ,[LIM(0,MAC_OctetArray[3],9) DTOS(MAC_OctetArray[3],MAC_StringArray[3]) ,LIM(10,MAC_OctetArray[3],15) [MOV(1,MAC_StringArray[3].LEN) ,CPT(MAC_StringArray[3].DATA[0],MAC_OctetArray[3]+55) ] ] ,[LIM(0,MAC_OctetArray[4],9) DTOS(MAC_OctetArray[4],MAC_StringArray[4]) ,LIM(10,MAC_OctetArray[4],15) [MOV(1,MAC_StringArray[4].LEN) ,CPT(MAC_StringArray[4].DATA[0],MAC_OctetArray[4]+55) ] ] ,[LIM(0,MAC_OctetArray[5],9) DTOS(MAC_OctetArray[5],MAC_StringArray[5]) ,LIM(10,MAC_OctetArray[5],15) [MOV(1,MAC_StringArray[5].LEN) ,CPT(MAC_StringArray[5].DATA[0],MAC_OctetArray[5]+55) ] ] ,[LIM(0,MAC_OctetArray[6],9) DTOS(MAC_OctetArray[6],MAC_StringArray[6]) ,LIM(10,MAC_OctetArray[6],15) [MOV(1,MAC_StringArray[6].LEN) ,CPT(MAC_StringArray[6].DATA[0],MAC_OctetArray[6]+55) ] ] ,[LIM(0,MAC_OctetArray[7],9) DTOS(MAC_OctetArray[7],MAC_StringArray[7]) ,LIM(10,MAC_OctetArray[7],15) [MOV(1,MAC_StringArray[7].LEN) ,CPT(MAC_StringArray[7].DATA[0],MAC_OctetArray[7]+55) ] ] ,[LIM(0,MAC_OctetArray[8],9) DTOS(MAC_OctetArray[8],MAC_StringArray[8]) ,LIM(10,MAC_OctetArray[8],15) [MOV(1,MAC_StringArray[8].LEN) ,CPT(MAC_StringArray[8].DATA[0],MAC_OctetArray[8]+55) ] ] ,[LIM(0,MAC_OctetArray[9],9) DTOS(MAC_OctetArray[9],MAC_StringArray[9]) ,LIM(10,MAC_OctetArray[9],15) [MOV(1,MAC_StringArray[9].LEN) ,CPT(MAC_StringArray[9].DATA[0],MAC_OctetArray[9]+55) ] ] ,[LIM(0,MAC_OctetArray[10],9) DTOS(MAC_OctetArray[10],MAC_StringArray[10]) ,LIM(10,MAC_OctetArray[10],15) [MOV(1,MAC_StringArray[10].LEN) ,CPT(MAC_StringArray[10].DATA[0],MAC_OctetArray[10]+55) ] ] ,[LIM(0,MAC_OctetArray[11],9) DTOS(MAC_OctetArray[11],MAC_StringArray[11]) ,LIM(10,MAC_OctetArray[11],15) [MOV(1,MAC_StringArray[11].LEN) ,CPT(MAC_StringArray[11].DATA[0],MAC_OctetArray[11]+55) ] ] ]MOV(1,punctuation_marks.LEN)MOV(45,punctuation_marks.DATA[0])[CONCAT(MAC_StringArray[10],Switch_Parameter.Switch_Data.MAC_Address,Switch_Parameter.Switch_Data.MAC_Address) CONCAT(MAC_StringArray[11],Switch_Parameter.Switch_Data.MAC_Address,Switch_Parameter.Switch_Data.MAC_Address) CONCAT(punctuation_marks,Switch_Parameter.Switch_Data.MAC_Address,Switch_Parameter.Switch_Data.MAC_Address) ,CONCAT(MAC_StringArray[8],Switch_Parameter.Switch_Data.MAC_Address,Switch_Parameter.Switch_Data.MAC_Address) CONCAT(MAC_StringArray[9],Switch_Parameter.Switch_Data.MAC_Address,Switch_Parameter.Switch_Data.MAC_Address) CONCAT(punctuation_marks,Switch_Parameter.Switch_Data.MAC_Address,Switch_Parameter.Switch_Data.MAC_Address) ,CONCAT(MAC_StringArray[6],Switch_Parameter.Switch_Data.MAC_Address,Switch_Parameter.Switch_Data.MAC_Address) CONCAT(MAC_StringArray[7],Switch_Parameter.Switch_Data.MAC_Address,Switch_Parameter.Switch_Data.MAC_Address) CONCAT(punctuation_marks,Switch_Parameter.Switch_Data.MAC_Address,Switch_Parameter.Switch_Data.MAC_Address) ,CONCAT(MAC_StringArray[4],Switch_Parameter.Switch_Data.MAC_Address,Switch_Parameter.Switch_Data.MAC_Address) CONCAT(MAC_StringArray[5],Switch_Parameter.Switch_Data.MAC_Address,Switch_Parameter.Switch_Data.MAC_Address) CONCAT(punctuation_marks,Switch_Parameter.Switch_Data.MAC_Address,Switch_Parameter.Switch_Data.MAC_Address) ,CONCAT(MAC_StringArray[2],Switch_Parameter.Switch_Data.MAC_Address,Switch_Parameter.Switch_Data.MAC_Address) CONCAT(MAC_StringArray[3],Switch_Parameter.Switch_Data.MAC_Address,Switch_Parameter.Switch_Data.MAC_Address) CONCAT(punctuation_marks,Switch_Parameter.Switch_Data.MAC_Address,Switch_Parameter.Switch_Data.MAC_Address) ,CONCAT(MAC_StringArray[0],Switch_Parameter.Switch_Data.MAC_Address,Switch_Parameter.Switch_Data.MAC_Address) CONCAT(MAC_StringArray[1],Switch_Parameter.Switch_Data.MAC_Address,Switch_Parameter.Switch_Data.MAC_Address) ];
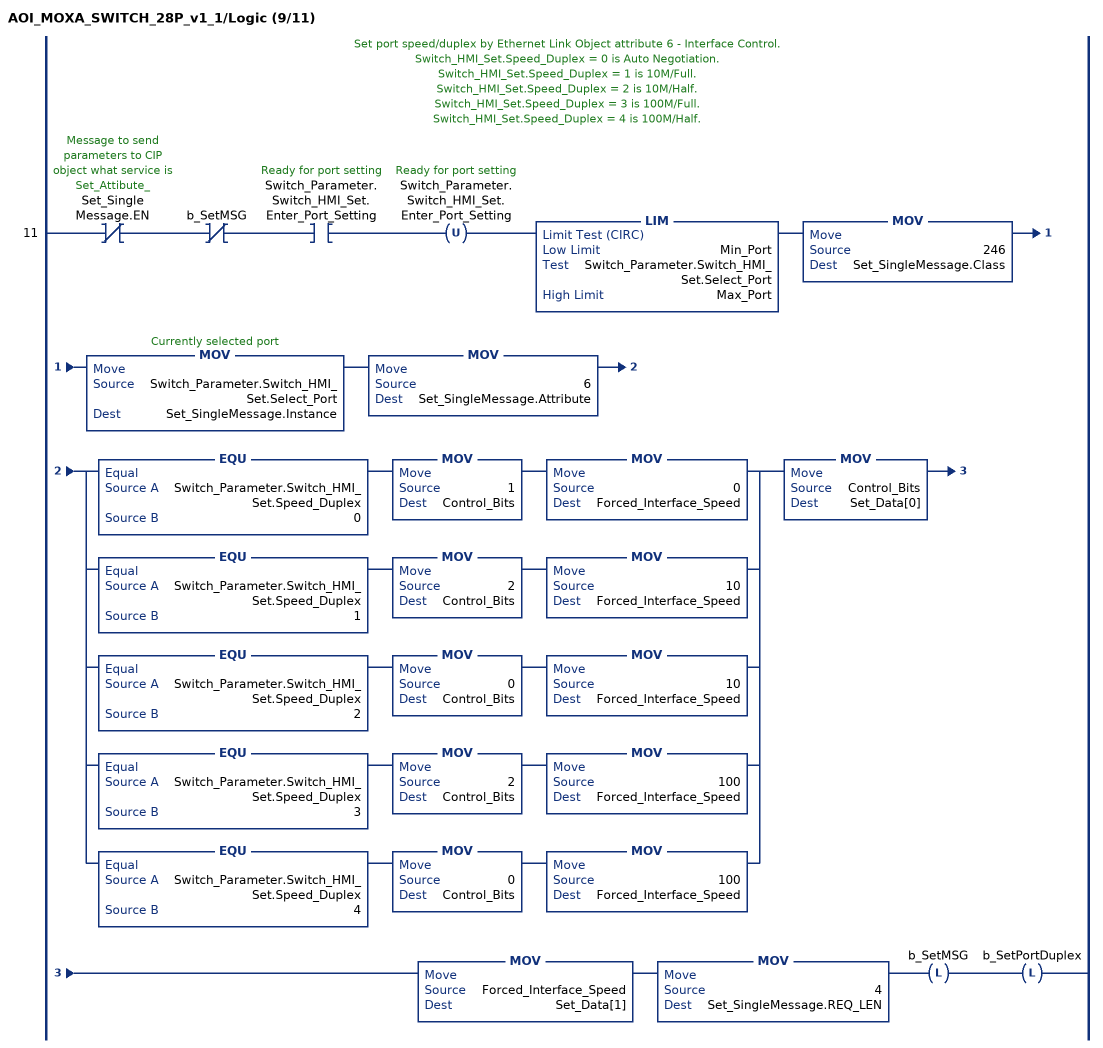
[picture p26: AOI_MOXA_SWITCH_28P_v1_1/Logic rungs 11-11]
   // Set port speed/duplex by Ethernet Link Object attribute 6 - Interface Control.
   // Switch_HMI_Set.Speed_Duplex = 0 is Auto Negotiation.
   // Switch_HMI_Set.Speed_Duplex = 1 is 10M/Full.
   // Switch_HMI_Set.Speed_Duplex = 2 is 10M/Half.
   // Switch_HMI_Set.Speed_Duplex = 3 is 100M/Full.
   // Switch_HMI_Set.Speed_Duplex = 4 is 100M/Half.
   11: XIO(Set_SingleMessage.EN)XIO(b_SetMSG)XIC(Switch_Parameter.Switch_HMI_Set.Enter_Port_Setting)OTU(Switch_Parameter.Switch_HMI_Set.Enter_Port_Setting)LIM(Min_Port,Switch_Parameter.Switch_HMI_Set.Select_Port,Max_Port)MOV(246,Set_SingleMessage.Class)MOV(Switch_Parameter.Switch_HMI_Set.Select_Port,Set_SingleMessage.Instance)MOV(6,Set_SingleMessage.Attribute)[EQU(Switch_Parameter.Switch_HMI_Set.Speed_Duplex,0) MOV(1,Control_Bits) MOV(0,Forced_Interface_Speed) ,EQU(Switch_Parameter.Switch_HMI_Set.Speed_Duplex,1) MOV(2,Control_Bits) MOV(10,Forced_Interface_Speed) ,EQU(Switch_Parameter.Switch_HMI_Set.Speed_Duplex,2) MOV(0,Control_Bits) MOV(10,Forced_Interface_Speed) ,EQU(Switch_Parameter.Switch_HMI_Set.Speed_Duplex,3) MOV(2,Control_Bits) MOV(100,Forced_Interface_Speed) ,EQU(Switch_Parameter.Switch_HMI_Set.Speed_Duplex,4) MOV(0,Control_Bits) MOV(100,Forced_Interface_Speed) ]MOV(Control_Bits,Set_Data[0])MOV(Forced_Interface_Speed,Set_Data[1])MOV(4,Set_SingleMessage.REQ_LEN)OTL(b_SetMSG)OTL(b_SetPortDuplex);
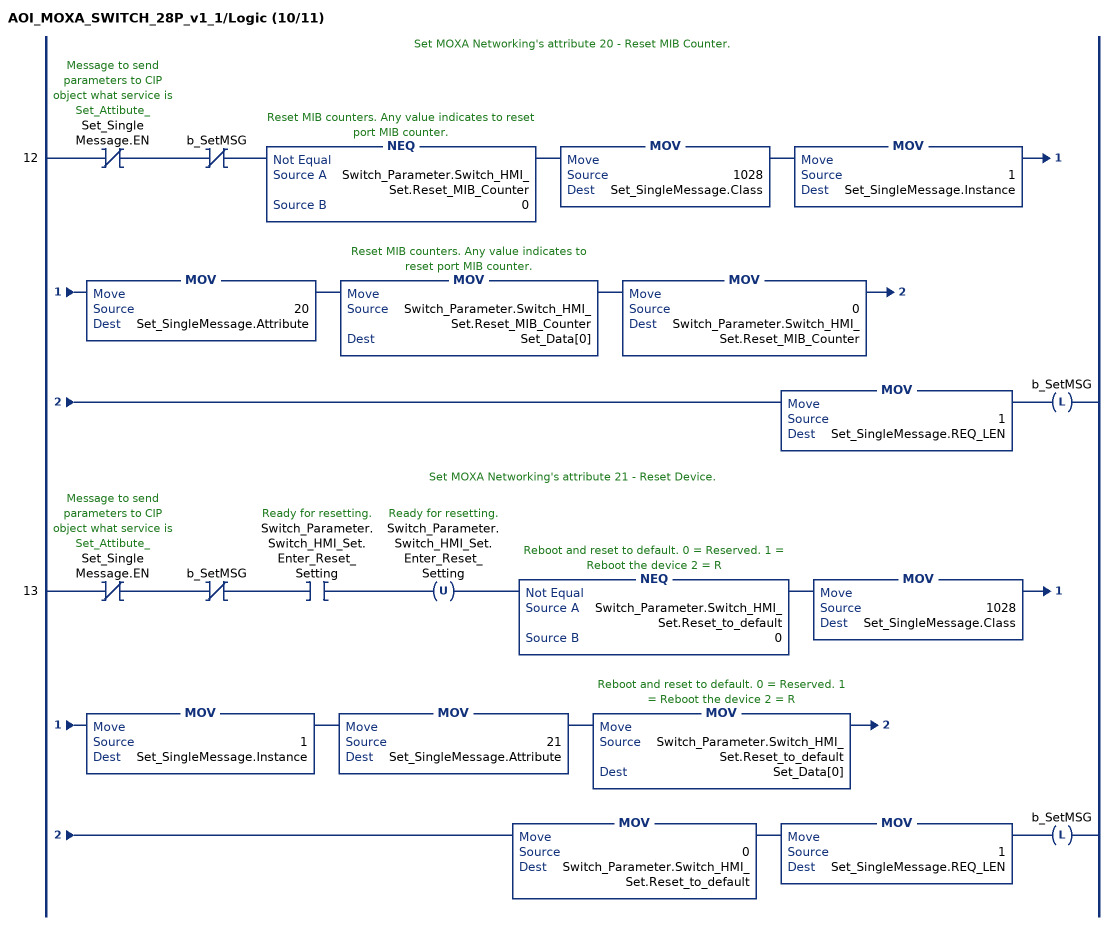
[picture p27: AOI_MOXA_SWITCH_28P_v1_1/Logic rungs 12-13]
   // Set MOXA Networking's attribute 20 - Reset MIB Counter.
   12: XIO(Set_SingleMessage.EN)XIO(b_SetMSG)NEQ(Switch_Parameter.Switch_HMI_Set.Reset_MIB_Counter,0)MOV(1028,Set_SingleMessage.Class)MOV(1,Set_SingleMessage.Instance)MOV(20,Set_SingleMessage.Attribute)MOV(Switch_Parameter.Switch_HMI_Set.Reset_MIB_Counter,Set_Data[0])MOV(0,Switch_Parameter.Switch_HMI_Set.Reset_MIB_Counter)MOV(1,Set_SingleMessage.REQ_LEN)OTL(b_SetMSG);
   // Set MOXA Networking's attribute 21 - Reset Device.
   13: XIO(Set_SingleMessage.EN)XIO(b_SetMSG)XIC(Switch_Parameter.Switch_HMI_Set.Enter_Reset_Setting)OTU(Switch_Parameter.Switch_HMI_Set.Enter_Reset_Setting)NEQ(Switch_Parameter.Switch_HMI_Set.Reset_to_default,0)MOV(1028,Set_SingleMessage.Class)MOV(1,Set_SingleMessage.Instance)MOV(21,Set_SingleMessage.Attribute)MOV(Switch_Parameter.Switch_HMI_Set.Reset_to_default,Set_Data[0])MOV(0,Switch_Parameter.Switch_HMI_Set.Reset_to_default)MOV(1,Set_SingleMessage.REQ_LEN)OTL(b_SetMSG);
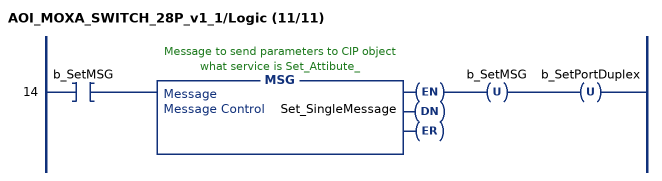
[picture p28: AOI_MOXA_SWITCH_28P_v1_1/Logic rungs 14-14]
   14: XIC(b_SetMSG)MSG(Set_SingleMessage)OTU(b_SetMSG)OTU(b_SetPortDuplex);
END_ROUTINE
END_ADD_ON_INSTRUCTION
